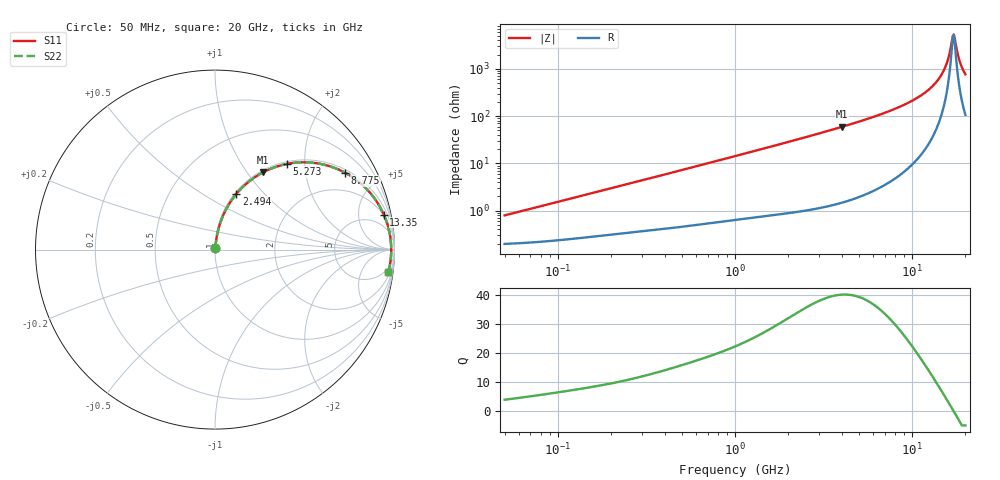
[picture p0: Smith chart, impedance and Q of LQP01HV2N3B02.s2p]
!Murata Part Number: LQP01HV2N3B02
!These Parameters are Measured in Series Mode Connection
!  o--[Z]--o
!Port1  Port2
!  o-------o
!Freq. Start=50[MHz] Stop=20[GHz], 401[Steps]
# Hz S RI R 50
!Freq.(Hz) S11(Real) S11(Imag) S21(Real) S21(Imag) S12(Real) S12(Imag) S22(Real) S22(Imag)
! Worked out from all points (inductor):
!   401 points, 50 MHz to 20 GHz, reference 50 ohm
!   read as one part in series: L = 2.44 nH near 51.52 MHz
!   highest Q = 40.2 at 4.027 GHz (marker M1), where L = 2.35 nH
!   self-resonance near 16.96 GHz
!   S11 on the Smith chart (normalised r, x): 50 MHz: 1.00, +0.02; 2.494 GHz: 1.02, +0.71; 5.273 GHz: 1.04, +1.62; 8.775 GHz: 1.12, +3.31; 13.35 GHz: 1.85, +9.36; 20 GHz: 3, -15
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5e7  0.00204 0.00768  0.998 -0.00768  0.998 -0.00768  0.00204 0.00768
1.364002e8  0.00307 0.0204  0.9969 -0.0204  0.9969 -0.0204  0.00307 0.0204
3.721004e8  0.00686 0.0534  0.9931 -0.0534  0.9931 -0.0534  0.00686 0.0534
1e9  0.0258 0.1376  0.9742 -0.1376  0.9742 -0.1376  0.0258 0.1376
2.493527e9  0.1193 0.3105  0.8807 -0.3105  0.8807 -0.3105  0.1193 0.3105
2.728004e9  0.1393 0.333  0.8607 -0.333  0.8607 -0.333  0.1393 0.333
4.026975e9  0.2661 0.4297  0.7339 -0.4297  0.7339 -0.4297  0.2661 0.4297
5.273168e9  0.3995 0.4771  0.6005 -0.4771  0.6005 -0.4771  0.3995 0.4771
7.442007e9  0.6162 0.4709  0.3838 -0.4709  0.3838 -0.4709  0.6162 0.4709
8.774992e9  0.7251 0.4283  0.2749 -0.4283  0.2749 -0.4283  0.7251 0.4283
1.115139e10  0.8653 0.3151  0.1347 -0.3151  0.1347 -0.3151  0.8653 0.3151
1.334722e10  0.9403 0.1955  0.0597 -0.1955  0.0597 -0.1955  0.9403 0.1955
1.438523e10  0.9611 0.1394  0.0389 -0.1394  0.0389 -0.1394  0.9611 0.1394
1.527346e10  0.9727 0.0926  0.0273 -0.0926  0.0273 -0.0926  0.9727 0.0926
1.597544e10  0.9784 0.0569  0.0216 -0.0569  0.0216 -0.0569  0.9784 0.0569
1.670968e10  0.9814 0.0207  0.0186 -0.0207  0.0186 -0.0207  0.9814 0.0207
1.696185e10  0.9818 0.00864  0.0182 -0.00864  0.0182 -0.00864  0.9818 0.00864
1.721783e10  0.9819 -0.00346  0.0181 0.00346  0.0181 0.00346  0.9819 -0.00346
1.747767e10  0.9817 -0.0156  0.0183 0.0156  0.0183 0.0156  0.9817 -0.0156
1.828096e10  0.9793 -0.0518  0.0207 0.0518  0.0207 0.0518  0.9793 -0.0518
1.88369e10  0.9762 -0.0758  0.0238 0.0758  0.0238 0.0758  0.9762 -0.0758
2e10  0.9666 -0.1231  0.0334 0.1231  0.0334 0.1231  0.9666 -0.1231
